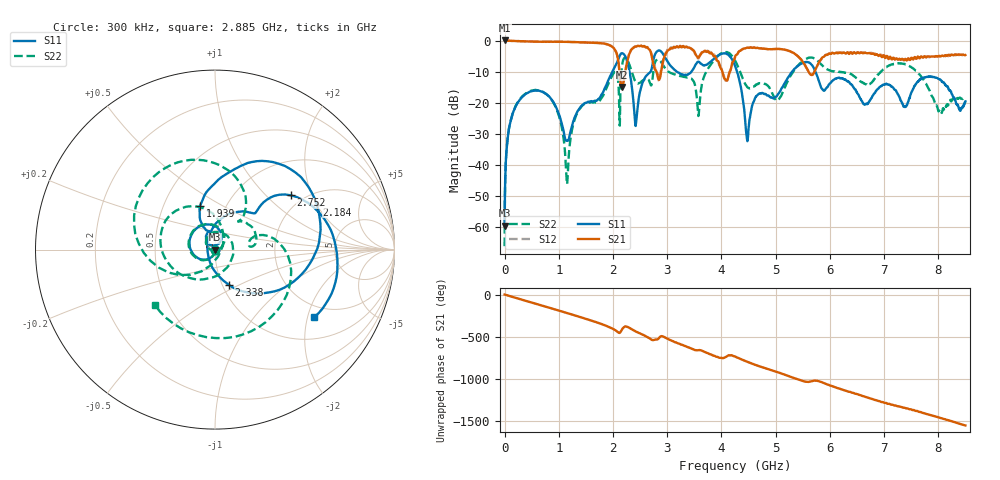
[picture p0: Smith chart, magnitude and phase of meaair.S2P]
!Agilent Technologies,E5071B,MY42402595,A.08.01
!Date: Mon Jan 01 23:26:48 2001
!Data & Calibration Information:
!Freq	S11:SOLT2(ON)	S21:SOLT2(ON)	S12:SOLT2(ON)	S22:SOLT2(ON)
# Hz S dB R 50
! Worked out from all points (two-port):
!   1601 points, 300 kHz to 8.5 GHz, reference 50 ohm
!   highest |S21| = 0.05 dB at 300 kHz (marker M1); lowest = -14.9 dB at 2.157 GHz (marker M2)
!   |S21| within 3 dB of the highest: start of sweep to 2.034 GHz; 4.371 GHz to 5.171 GHz (799.5 MHz wide, 16.8 % of centre)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
!   lowest |S11| = -59.7 dB at 300 kHz (marker M3), VSWR 1.00, Z = 50.1 - j0.0815 ohm
!   |S11| at or under -10 dB: start of sweep to 1.987 GHz; 4.289 GHz to 5.304 GHz (1.015 GHz wide, 21.2 % of centre); 5.732 GHz to end of sweep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
!   |S22| runs from -66.2 to -3.7 dB; largest |S21 - S12| = 0.069
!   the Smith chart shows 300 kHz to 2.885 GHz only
!   S11 on the Smith chart (normalised r, x): 300 kHz: 1.00, -0.00; 1.939 GHz: 0.76, +0.40; 2.184 GHz: 2.46, +2.00; 2.338 GHz: 1.07, -0.44; 2.752 GHz: 1.72, +1.43; 2.885 GHz: 1.62, -2.21
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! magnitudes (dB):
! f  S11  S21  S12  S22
! 300 kHz  -59.7  0.1  0.0  -66.2
! 74.67 MHz  -29.1  0.0  0.0  -29.0
! 276.5 MHz  -19.2  -0.2  -0.2  -18.9
! 860.9 MHz  -18.9  -0.3  -0.4  -18.9
! 1.153 GHz  -32.3  -0.4  -0.4  -46.3
! 1.419 GHz  -21.0  -0.6  -0.6  -21.2
! 1.939 GHz  -11.8  -1.5  -1.6  -12.9
! 2.157 GHz  -4.1  -14.9  -14.8  -9.7
! 2.184 GHz  -4.2  -14.0  -14.2  -6.5
! 2.338 GHz  -13.5  -2.9  -3.0  -9.7
! 2.428 GHz  -26.0  -1.9  -1.8  -13.5
! 2.752 GHz  -5.7  -8.2  -8.3  -8.8
! 2.837 GHz  -3.2  -12.4  -11.8  -6.1
! 2.885 GHz  -3.5  -10.2  -9.0  -6.8
! 3.575 GHz  -6.8  -5.5  -5.8  -24.3
! 4.25 GHz  -8.1  -5.3  -5.5  -6.4
! 4.479 GHz  -32.4  -2.2  -2.3  -15.0
! 5.042 GHz  -17.3  -2.7  -2.7  -19.3
! 5.669 GHz  -7.9  -11.1  -11.1  -5.5
! 6.646 GHz  -20.6  -3.9  -3.8  -13.9
! 7.087 GHz  -14.2  -5.9  -5.3  -8.1
! 8.5 GHz  -19.6  -4.7  -4.7  -19.8
